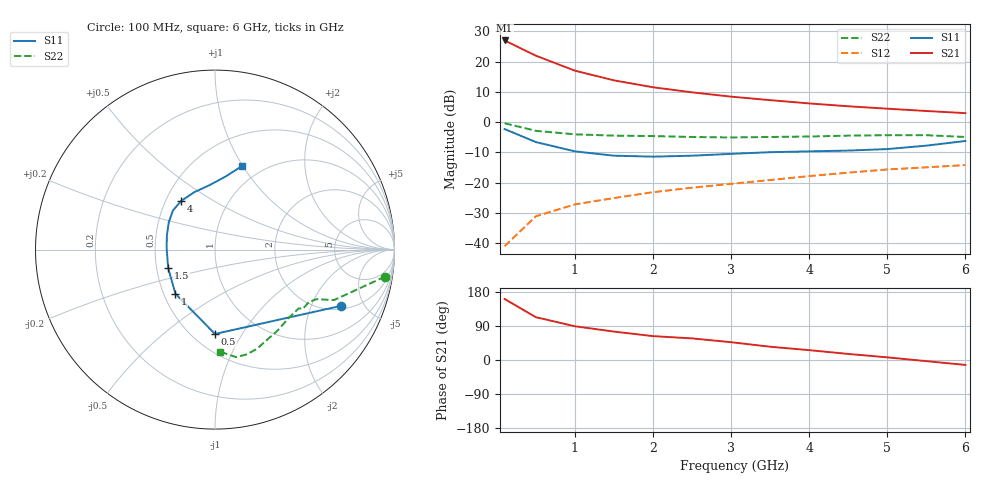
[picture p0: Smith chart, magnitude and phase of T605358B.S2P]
!AT-60535
!S-PARAMETERS at Vce=8V  Ic=10mA.  LAST UPDATED 07-21-92
!OBSOLETED Feb 1994 - nearest replacement: AT-41435
# ghz s ma r 50
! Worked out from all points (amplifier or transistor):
!   13 points, 100 MHz to 6 GHz, reference 50 ohm
!   highest |S21| = 27.0 dB at 100 MHz (marker M1)
!   |S21| within 3 dB of that: start of sweep to 338.8 MHz
!   unconditionally stable (mu >= 1): 1.296 GHz to 4.491 GHz
!   at 1 GHz: K = 0.89, MSG = 22.1 dB, |S12| = -27.1 dB
!   at 3 GHz: K = 1.19, MAG = 11.7 dB, |S12| = -20.4 dB
!   at 6 GHz: K = 0.85, MSG = 8.6 dB, |S12| = -14.2 dB
!   S11 on the Smith chart (normalised r, x): 100 MHz: 2.19, -3.37; 500 MHz: 0.64, -0.77; 1 GHz: 0.57, -0.32; 1.5 GHz: 0.58, -0.13; 4 GHz: 0.60, +0.36; 6 GHz: 0.81, +0.99
0.1  0.77 -24.0  22.31 161.0  0.009 76.0  0.96 -9.0
0.5  0.47 -90.0  12.51 113.0  0.028 59.0  0.72 -23.0
1  0.33 -132.0  7.08 89.0  0.044 61.0  0.63 -26.0
1.5  0.28 -159.0  4.9 75.0  0.056 58.0  0.6 -29.0
2  0.27 177.0  3.77 63.0  0.07 58.0  0.59 -34.0
2.5  0.28 163.0  3.11 57.0  0.083 63.0  0.57 -35.0
3  0.3 149.0  2.64 47.0  0.096 60.0  0.56 -43.0
3.5  0.32 137.0  2.31 35.0  0.111 58.0  0.57 -52.0
4  0.33 125.0  2.04 26.0  0.129 54.0  0.58 -60.0
4.5  0.34 110.0  1.83 16.0  0.147 50.0  0.6 -67.0
5  0.36 95.0  1.67 7.0  0.166 46.0  0.61 -73.0
5.5  0.41 82.0  1.53 -3.0  0.18 40.0  0.61 -79.0
6  0.49 72.0  1.41 -13.0  0.196 37.0  0.57 -87.0
